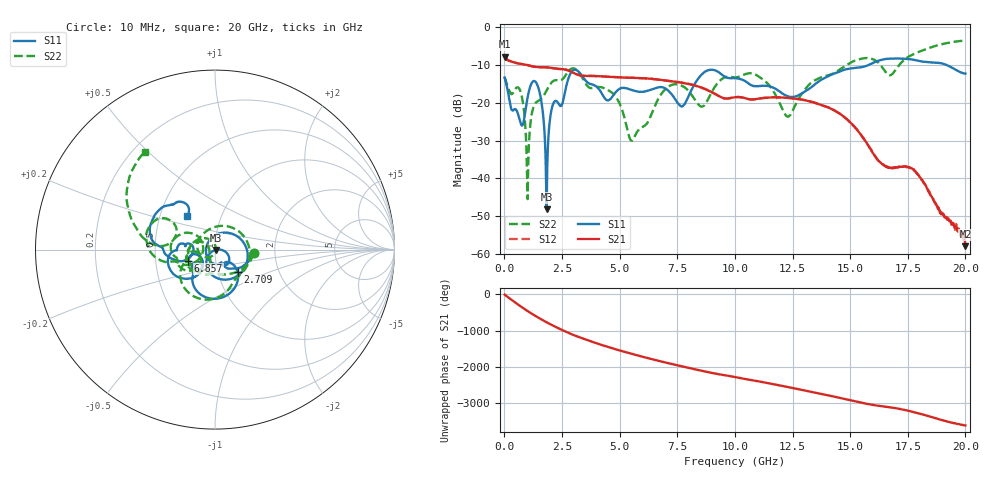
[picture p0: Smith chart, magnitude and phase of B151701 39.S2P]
!  2-Port S-parameters saved by WinCal
! VAR MeasName=S-Parameters (CALIBRATED_DATA) read from VNA (N5244A)
! VAR MeasDate=2015-12-24 19:13:57
! VAR NAME=B151701 39
! VAR FILENAME=B151701 39.S2P
! VAR DATE=2015-12-24 19:13:57
! VAR PHYS_PORTS=1,3
# Hz S DB R 50
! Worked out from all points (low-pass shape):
!   801 points, 10 MHz to 20 GHz, reference 50 ohm
!   highest |S21| = -7.79 dB at 10 MHz (marker M1); lowest = -58.0 dB at 20 GHz (marker M2)
!   |S21| within 3 dB of the highest: start of sweep to 2.101 GHz
!   lowest |S11| = -48.2 dB at 1.834 GHz (marker M3), VSWR 1.01, Z = 50.3 - j0.208 ohm
!   |S11| at or under -10 dB: start of sweep to 15.79 GHz; 19.18 GHz to end of sweep
!   |S22| runs from -45.5 to -3.5 dB; largest |S21 - S12| = 0.0012
!   S11 on the Smith chart (normalised r, x): 10 MHz: 1.55, -0.06; 2.709 GHz: 1.24, -0.32; 6.857 GHz: 0.74, -0.09; 20 GHz: 0.69, +0.27
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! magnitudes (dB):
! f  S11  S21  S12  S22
! 10 MHz  -13.3  -7.8  -7.8  -13.2
! 709.6 MHz  -25.4  -9.7  -9.7  -17.2
! 1.01 GHz  -18.5  -10.0  -10.0  -45.5
! 1.459 GHz  -15.7  -10.5  -10.5  -19.5
! 1.834 GHz  -48.2  -10.6  -10.6  -16.7
! 2.084 GHz  -20.9  -10.8  -10.8  -14.4
! 2.709 GHz  -15.0  -11.3  -11.3  -12.2
! 3.358 GHz  -12.7  -12.8  -12.8  -13.1
! 4.808 GHz  -17.3  -13.2  -13.2  -18.2
! 5.507 GHz  -16.5  -13.4  -13.4  -30.0
! 6.682 GHz  -15.9  -13.8  -13.8  -18.9
! 6.857 GHz  -15.9  -14.0  -14.0  -17.2
! 7.706 GHz  -21.0  -14.7  -14.7  -15.5
! 8.581 GHz  -12.4  -16.0  -16.0  -21.0
! 10.01 GHz  -13.5  -18.5  -18.5  -13.3
! 11.2 GHz  -15.5  -18.8  -18.7  -13.7
! 12.3 GHz  -18.3  -18.7  -18.7  -23.7
! 13.35 GHz  -15.7  -19.8  -19.8  -14.5
! 15.63 GHz  -10.4  -29.8  -29.8  -8.2
! 16.68 GHz  -8.3  -37.2  -37.1  -12.7
! 17.8 GHz  -8.6  -38.0  -38.0  -7.0
! 20 GHz  -12.2  -58.0  -55.6  -3.5
